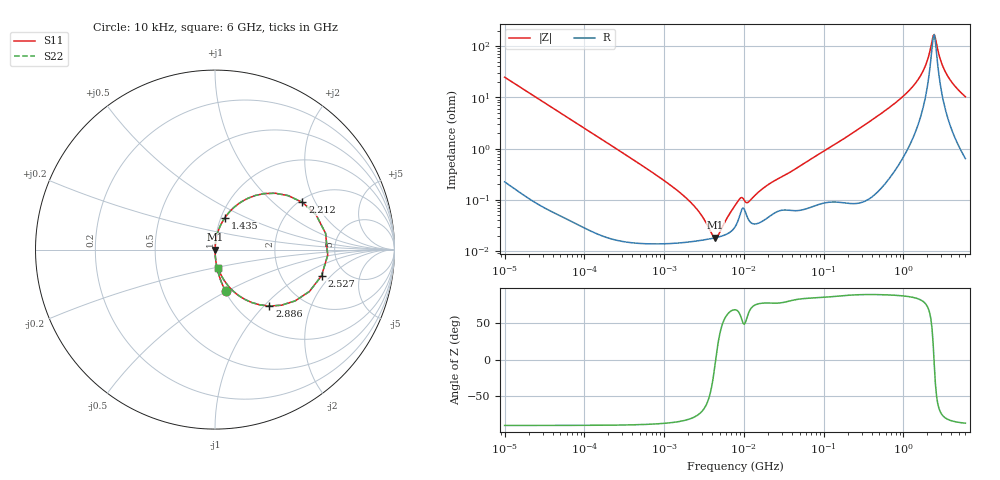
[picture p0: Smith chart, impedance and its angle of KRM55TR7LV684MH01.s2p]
!Murata Part Number: KRM55TR7LV684MH01
!These Parameters are Measured in Series Mode Connection
!Data Generated on Jan 08, 2026
!  o--ll--o
!Port1  Port2
!  o------o
!Operation Temp=25[degC], DC Bias Voltage=0[V]
!Freq. Start=10[kHz] Stop=6[GHz] 401[Steps]
# Hz S RI R 50
!Freq.(Hz) S11(Real) S11(Imag) S21(Real) S21(Imag) S12(Real) S12(Imag) S22(Real) S22(Imag)
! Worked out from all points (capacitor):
!   401 points, 10 kHz to 6 GHz, reference 50 ohm
!   read as one part in series: C = 642 nF near 10.69 kHz
!   lowest |Z| = 18.3 mohm at 4.401 MHz (marker M1)
!   series resonance near 4.442 MHz, so ESL is about 2 nH
!   S11 on the Smith chart (normalised r, x): 10 kHz: 1.00, -0.49; 1.435 GHz: 1.04, +0.38; 2.212 GHz: 2.09, +1.59; 2.527 GHz: 3.36, -1.57; 2.886 GHz: 1.39, -1.08; 6 GHz: 1.01, -0.21
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10000  0.0595 -0.2321  0.9405 0.2321  0.9405 0.2321  0.0595 -0.2321
26237  0.00969 -0.0937  0.9903 0.0937  0.9903 0.0937  0.00969 -0.0937
92862  0.00102 -0.0269  0.999 0.0269  0.999 0.0269  0.00102 -0.0269
862344  0.000146 -0.0028  0.9999 0.0028  0.9999 0.0028  0.000146 -0.0028
2262542  0.000154 -0.000814  0.9998 0.000814  0.9998 0.000814  0.000154 -0.000814
4400522  0.000183 -1.05e-05  0.9998 1.05e-05  0.9998 1.05e-05  0.000183 -1.05e-05
4862284  0.00019 0.000103  0.9998 -0.000103  0.9998 -0.000103  0.00019 0.000103
7745967  0.000297 0.000717  0.9997 -0.000717  0.9997 -0.000717  0.000297 0.000717
9147502  0.000574 0.000934  0.9994 -0.000934  0.9994 -0.000934  0.000574 0.000934
1.15457e7  0.000403 0.000828  0.9996 -0.000828  0.9996 -0.000828  0.000403 0.000828
2.032318e7  0.000463 0.00194  0.9995 -0.00194  0.9995 -0.00194  0.000463 0.00194
7.193098e7  0.000775 0.00643  0.9992 -0.00643  0.9992 -0.00643  0.000775 0.00643
6.67969e8  0.00658 0.0627  0.9934 -0.0627  0.9934 -0.0627  0.00658 0.0627
1.435489e9  0.0551 0.1775  0.9449 -0.1775  0.9449 -0.1775  0.0551 0.1775
1.873109e9  0.1872 0.2876  0.8128 -0.2876  0.8128 -0.2876  0.1872 0.2876
2.212024e9  0.4875 0.2631  0.5125 -0.2631  0.5125 -0.2631  0.4875 0.2631
2.364181e9  0.6163 0.0903  0.3837 -0.0903  0.3837 -0.0903  0.6163 0.0903
2.526803e9  0.5936 -0.1461  0.4064 0.1461  0.4064 0.1461  0.5936 -0.1461
2.700612e9  0.4467 -0.2858  0.5533 0.2858  0.5533 0.2858  0.4467 -0.2858
2.886376e9  0.3035 -0.3145  0.6965 0.3145  0.6965 0.3145  0.3035 -0.3145
3.643096e9  0.0886 -0.2188  0.9114 0.2188  0.9114 0.2188  0.0886 -0.2188
6e9  0.0166 -0.1003  0.9834 0.1003  0.9834 0.1003  0.0166 -0.1003
